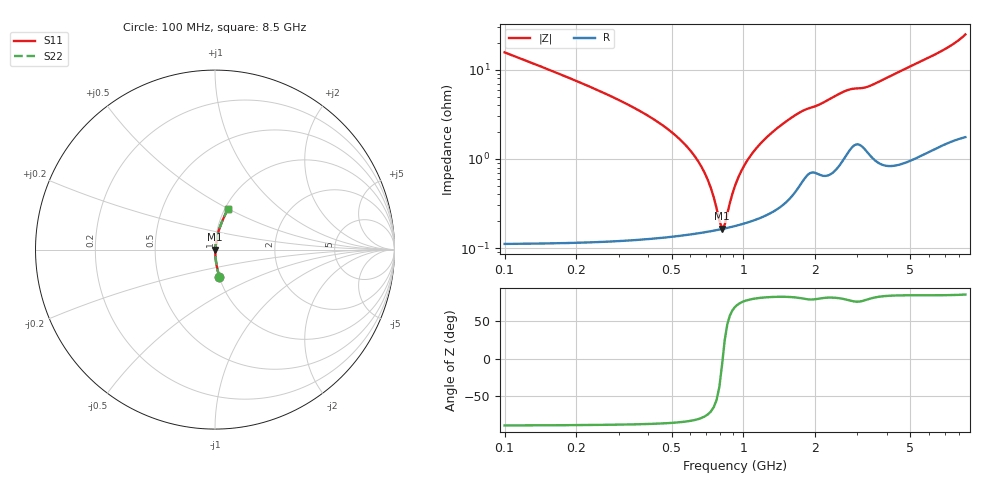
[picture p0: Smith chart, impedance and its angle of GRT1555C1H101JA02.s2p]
!Murata Part Number: GRT1555C1H101JA02
!These Parameters are Measured in Series Mode Connection
!Data Generated on Jun 19, 2026
!  o--ll--o
!Port1  Port2
!  o------o
!Operation Temp=25[degC], DC Bias Voltage=0[V]
!Freq. Start=100[MHz] Stop=9[GHz] 401[Steps]
# Hz S RI R 50
!Freq.(Hz) S11(Real) S11(Imag) S21(Real) S21(Imag) S12(Real) S12(Imag) S22(Real) S22(Imag)
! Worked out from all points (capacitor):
!   401 points, 100 MHz to 8.5 GHz, reference 50 ohm
!   read as one part in series: C = 100 pF near 142 MHz
!   lowest |Z| = 165 mohm at 814 MHz (marker M1)
!   series resonance near 818.8 MHz, so ESL is about 380 pH
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1e8  0.025 -0.1527  0.975 0.1527  0.975 0.1527  0.025 -0.1527
2.47e8  0.00457 -0.0582  0.9954 0.0582  0.9954 0.0582  0.00457 -0.0582
5.2e8  0.00168 -0.0182  0.9983 0.0182  0.9983 0.0182  0.00168 -0.0182
6.25e8  0.00155 -0.0106  0.9984 0.0106  0.9984 0.0106  0.00155 -0.0106
6.88e8  0.00155 -0.00679  0.9985 0.00679  0.9985 0.00679  0.00155 -0.00679
7.72e8  0.00159 -0.00229  0.9984 0.00229  0.9984 0.00229  0.00159 -0.00229
8.14e8  0.00163 -0.000225  0.9984 0.000225  0.9984 0.000225  0.00163 -0.000225
8.35e8  0.00166 0.000766  0.9983 -0.000766  0.9983 -0.000766  0.00166 0.000766
8.56e8  0.00168 0.00173  0.9983 -0.00173  0.9983 -0.00173  0.00168 0.00173
9.19e8  0.00178 0.00451  0.9982 -0.00451  0.9982 -0.00451  0.00178 0.00451
9.61e8  0.00185 0.00628  0.9981 -0.00628  0.9981 -0.00628  0.00185 0.00628
1.066e9  0.00208 0.0104  0.9979 -0.0104  0.9979 -0.0104  0.00208 0.0104
1.255e9  0.00265 0.0173  0.9974 -0.0173  0.9974 -0.0173  0.00265 0.0173
1.507e9  0.00391 0.0259  0.9961 -0.0259  0.9961 -0.0259  0.00391 0.0259
1.822e9  0.00742 0.0348  0.9926 -0.0348  0.9926 -0.0348  0.00742 0.0348
2.578e9  0.0119 0.0535  0.9881 -0.0535  0.9881 -0.0535  0.0119 0.0535
2.914e9  0.0174 0.058  0.9826 -0.058  0.9826 -0.058  0.0174 0.058
3.313e9  0.0155 0.0617  0.9845 -0.0617  0.9845 -0.0617  0.0155 0.0617
4.3e9  0.0161 0.0873  0.9839 -0.0873  0.9839 -0.0873  0.0161 0.0873
5.707e9  0.0268 0.1237  0.9732 -0.1237  0.9732 -0.1237  0.0268 0.1237
7.114e9  0.0432 0.1651  0.9568 -0.1651  0.9568 -0.1651  0.0432 0.1651
8.5e9  0.0725 0.2264  0.9275 -0.2264  0.9275 -0.2264  0.0725 0.2264
